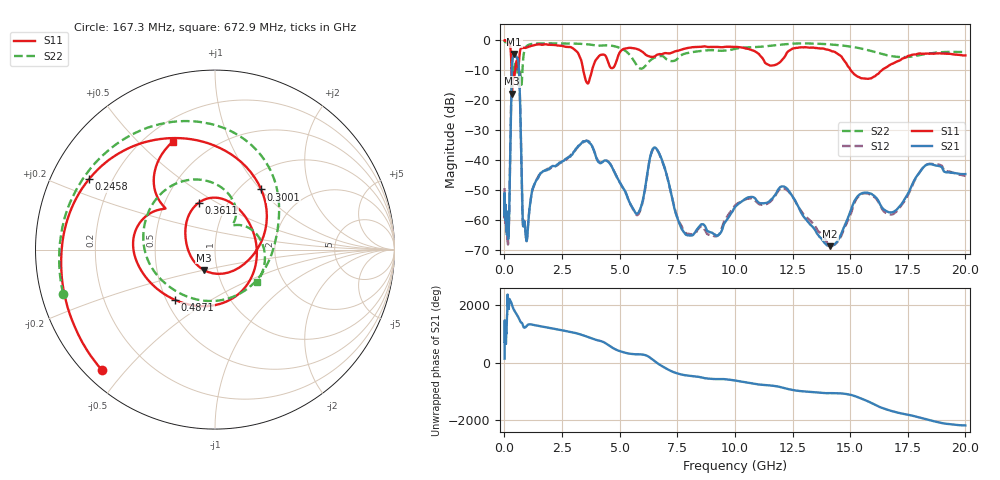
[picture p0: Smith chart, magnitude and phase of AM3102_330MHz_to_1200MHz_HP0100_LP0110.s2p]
! Date/Time: Tue, Sep 11, 2018 5:12 PM
! Network Analyzer: Agilent Technologies E8362B Rev: A.07.50.63
! Sweep from 0.010 to 20.000 GHz, 1601 Points, Sweep Type: LOG
! Power Supply: 4.949 V, 0.001 A
# Hz S DB R 50
!freq MagS11 AngS11 MagS21 AngS21 MagS12 AngS12 MagS22 AngS22
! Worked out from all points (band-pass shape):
!   1601 points, 10 MHz to 20 GHz, reference 50 ohm
!   highest |S21| = -4.55 dB at 426.5 MHz (marker M1); lowest = -68.8 dB at 14.14 GHz (marker M2)
!   |S21| within 3 dB of the highest: 337.3 MHz to 611 MHz (273.7 MHz wide, 57.7 % of centre)
!   lowest |S11| = -17.7 dB at 330 MHz (marker M3), VSWR 1.30, Z = 43 - j9.89 ohm
!   |S11| at or under -10 dB: 307.7 MHz to 468.5 MHz (160.9 MHz wide, 41.5 % of centre); 3.423 GHz to 3.803 GHz (379.9 MHz wide, 10.5 % of centre); 15.03 GHz to 16.37 GHz (1.343 GHz wide, 8.55 % of centre)
!   |S22| runs from -15.6 to -0.2 dB; largest |S21 - S12| = 0.0095
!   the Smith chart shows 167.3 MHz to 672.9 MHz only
!   S11 on the Smith chart (normalised r, x): 167.3 MHz: 0.05, -0.43; 245.8 MHz: 0.12, +0.26; 300.1 MHz: 1.24, +1.01; 361.1 MHz: 0.74, +0.42; 487.1 MHz: 0.56, -0.36; 672.9 MHz: 0.31, +0.64
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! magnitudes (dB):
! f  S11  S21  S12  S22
! 10 MHz  0.0  -51.7  -49.3  -0.2
! 35.55 MHz  0.0  -59.2  -56.7  -0.4
! 126.4 MHz  -0.4  -61.9  -60.5  -0.9
! 167.3 MHz  -0.7  -66.2  -64.9  -1.1
! 245.8 MHz  -1.9  -41.7  -41.6  -1.9
! 300.1 MHz  -7.5  -16.8  -16.9  -4.1
! 330 MHz  -17.7  -8.6  -8.6  -8.0
! 361.1 MHz  -11.2  -5.9  -5.9  -10.8
! 426.5 MHz  -12.4  -4.5  -4.6  -9.3
! 447.2 MHz  -11.2  -4.6  -4.6  -8.5
! 487.1 MHz  -8.9  -4.9  -5.0  -7.5
! 672.9 MHz  -3.8  -18.3  -18.4  -10.6
! 794.6 MHz  -2.5  -59.8  -60.6  -8.3
! 947.3 MHz  -2.4  -66.5  -67.0  -2.1
! 1.59 GHz  -1.4  -44.2  -44.2  -1.0
! 3.599 GHz  -14.3  -33.7  -33.5  -1.3
! 5.652 GHz  -2.6  -57.2  -57.4  -7.2
! 6.58 GHz  -5.0  -36.0  -36.2  -5.6
! 7.92 GHz  -2.6  -65.1  -64.6  -4.2
! 12.09 GHz  -6.1  -48.8  -49.3  -1.3
! 14.14 GHz  -3.4  -68.8  -68.3  -1.3
! 20 GHz  -5.0  -44.7  -45.3  -3.9
